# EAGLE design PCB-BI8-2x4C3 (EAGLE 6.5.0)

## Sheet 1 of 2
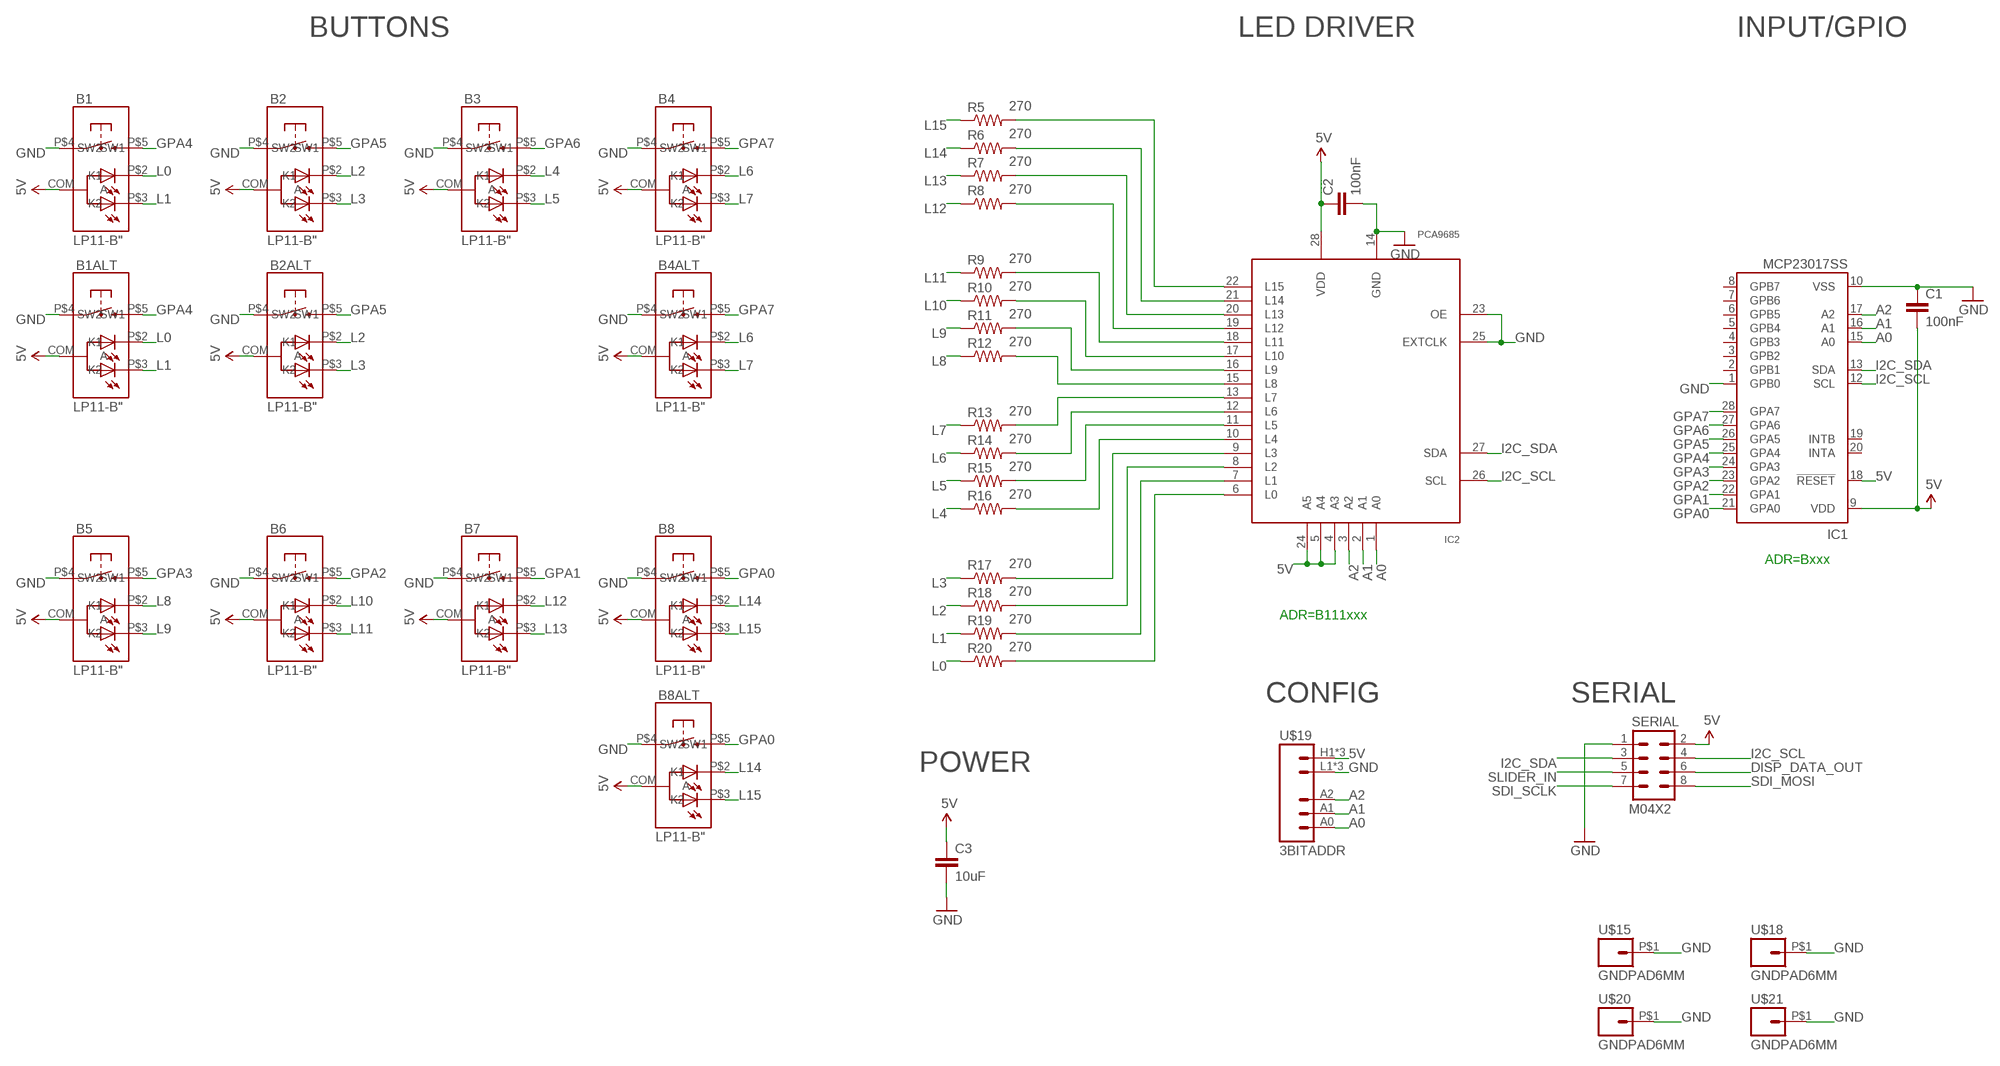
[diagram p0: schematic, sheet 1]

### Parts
B1  LP11-B"  [LP11]
B1ALT  LP11-B"  [LP11]
B2  LP11-B"  [LP11]
B2ALT  LP11-B"  [LP11]
B3  LP11-B"  [LP11]
B4  LP11-B"  [LP11]
B4ALT  LP11-B"  [LP11]
B5  LP11-B"  [LP11]
B6  LP11-B"  [LP11]
B7  LP11-B"  [LP11]
B8  LP11-B"  [LP11]
B8ALT  LP11-B"  [LP11]
C1  100nF  CAP0603-CAP  [0603-CAP]
C2  100nF  CAP0603-CAP  [0603-CAP]
C3  10uF  CAP0805  [0805]
IC1  MCP23017SS  [SSOP28]
IC2  PCA9685  [TSSOP28]
R5  270  RESISTOR0603-RES  [0603-RES]
R6  270  RESISTOR0603-RES  [0603-RES]
R7  270  RESISTOR0603-RES  [0603-RES]
R8  270  RESISTOR0603-RES  [0603-RES]
R9  270  RESISTOR0603-RES  [0603-RES]
R10  270  RESISTOR0603-RES  [0603-RES]
R11  270  RESISTOR0603-RES  [0603-RES]
R12  270  RESISTOR0603-RES  [0603-RES]
R13  270  RESISTOR0603-RES  [0603-RES]
R14  270  RESISTOR0603-RES  [0603-RES]
R15  270  RESISTOR0603-RES  [0603-RES]
R16  270  RESISTOR0603-RES  [0603-RES]
R17  270  RESISTOR0603-RES  [0603-RES]
R18  270  RESISTOR0603-RES  [0603-RES]
R19  270  RESISTOR0603-RES  [0603-RES]
R20  270  RESISTOR0603-RES  [0603-RES]
SERIAL  M04X2  [2X4]
U$15  GNDPAD6MM  [3.2MMPAD6MM]
U$18  GNDPAD6MM  [3.2MMPAD6MM]
U$19  3BITADDR  [3BITADDR]
U$20  GNDPAD6MM  [3.2MMPAD6MM]
U$21  GNDPAD6MM  [3.2MMPAD6MM]

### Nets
5V [Power]: B1.COM(A) B1ALT.COM(A) B2.COM(A) B2ALT.COM(A) B3.COM(A) B4.COM(A) B4ALT.COM(A) B5.COM(A) B6.COM(A) B7.COM(A) B8.COM(A) B8ALT.COM(A) C1.2 C2.1 C3.1 IC1.9(VDD) IC1.18(!RESET) IC2.4(A3) IC2.5(A4) IC2.24(A5) IC2.28(VDD) SERIAL.2 U$19.H1(VCC) U$19.H2(VCC) U$19.H3(VCC)
A0: IC1.15(A0) IC2.1(A0) U$19.A0
A1: IC1.16(A1) IC2.2(A1) U$19.A1
A2: IC1.17(A2) IC2.3(A2) U$19.A2
DISP_DATA_OUT: SERIAL.6
GND [Power]: B1.P$4(SW1) B1ALT.P$4(SW1) B2.P$4(SW1) B2ALT.P$4(SW1) B3.P$4(SW1) B4.P$4(SW1) B4ALT.P$4(SW1) B5.P$4(SW1) B6.P$4(SW1) B7.P$4(SW1) B8.P$4(SW1) B8ALT.P$4(SW1) C1.1 C2.2 C3.2 IC1.1(GPB0) IC1.10(VSS) IC2.14(GND) IC2.23(OE) IC2.25(EXTCLK) SERIAL.1 U$15.P$1 U$18.P$1 U$19.L1(GND) U$19.L2(GND) U$19.L3(GND) U$20.P$1 U$21.P$1
GPA0: B8.P$5(SW2) B8ALT.P$5(SW2) IC1.21(GPA0)
GPA1: B7.P$5(SW2) IC1.22(GPA1)
GPA2: B6.P$5(SW2) IC1.23(GPA2)
GPA3: B5.P$5(SW2) IC1.24(GPA3)
GPA4: B1.P$5(SW2) B1ALT.P$5(SW2) IC1.25(GPA4)
GPA5: B2.P$5(SW2) B2ALT.P$5(SW2) IC1.26(GPA5)
GPA6: B3.P$5(SW2) IC1.27(GPA6)
GPA7: B4.P$5(SW2) B4ALT.P$5(SW2) IC1.28(GPA7)
I2C_SCL: IC1.12(SCL) IC2.26(SCL) SERIAL.4
I2C_SDA: IC1.13(SDA) IC2.27(SDA) SERIAL.3
L0: B1.P$2(K1) B1ALT.P$2(K1) R20.1
L1: B1.P$3(K2) B1ALT.P$3(K2) R19.1
L2: B2.P$2(K1) B2ALT.P$2(K1) R18.1
L3: B2.P$3(K2) B2ALT.P$3(K2) R17.1
L4: B3.P$2(K1) R16.1
L5: B3.P$3(K2) R15.1
L6: B4.P$2(K1) B4ALT.P$2(K1) R14.1
L7: B4.P$3(K2) B4ALT.P$3(K2) R13.1
L8: B5.P$2(K1) R12.1
L9: B5.P$3(K2) R11.1
L10: B6.P$2(K1) R10.1
L11: B6.P$3(K2) R9.1
L12: B7.P$2(K1) R8.1
L13: B7.P$3(K2) R7.1
L14: B8.P$2(K1) B8ALT.P$2(K1) R6.1
L15: B8.P$3(K2) B8ALT.P$3(K2) R5.1
N$4: IC2.13(L7) R13.2
N$5: IC2.12(L6) R14.2
N$7: IC2.11(L5) R15.2
N$9: IC2.10(L4) R16.2
N$10: IC2.9(L3) R17.2
N$11: IC2.8(L2) R18.2
N$12: IC2.7(L1) R19.2
N$19: IC2.6(L0) R20.2
N$20: IC2.15(L8) R12.2
N$21: IC2.16(L9) R11.2
N$22: IC2.17(L10) R10.2
N$23: IC2.18(L11) R9.2
N$24: IC2.19(L12) R8.2
N$25: IC2.20(L13) R7.2
N$26: IC2.21(L14) R6.2
N$27: IC2.22(L15) R5.2
SDI_MOSI: SERIAL.8
SDI_SCLK: SERIAL.7
SLIDER_IN: SERIAL.5
Unconnected: IC1.2(GPB1) IC1.3(GPB2) IC1.4(GPB3) IC1.5(GPB4) IC1.6(GPB5) IC1.7(GPB6) IC1.8(GPB7) IC1.19(INTB) IC1.20(INTA)

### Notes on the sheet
- BUTTONS | LED DRIVER | INPUT/GPIO
- ADR=Bxxx
- ADR=B111xxx
- CONFIG | SERIAL
- POWER

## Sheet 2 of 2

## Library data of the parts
B1 B1ALT B2 B2ALT B3 B4 B4ALT B5-B8 B8ALT = SKAARHOJ:LP11-B
C1-C3 = SparkFun:CAP: Capacitor
IC1 = microchip:MCP23017: http://ww1.microchip.com/downloads/en/DeviceDoc/21952a.pdf Source: http://ww1.microchip.com/downloads/en/DeviceDoc/21952a.pdf; MF: MICROCHIP; MPN: MCP23017-E/SS; OC_FARNELL: 1467674; OC_NEWARK: 31K2960
IC2 = wsmith:PCA9685
R5-R20 = SparkFun:RESISTOR: Resistor
SERIAL = SparkFun:M04X2
U$15 U$18 U$20 U$21 = SKAARHOJ:GNDPAD
U$19 = SKAARHOJ:3BITADDR

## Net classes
0 default: width 0.203 mm, drill 0.406 mm, clearance 0.203 mm
1 Power: width 0.406 mm, drill 0.61 mm, clearance 0.203 mm

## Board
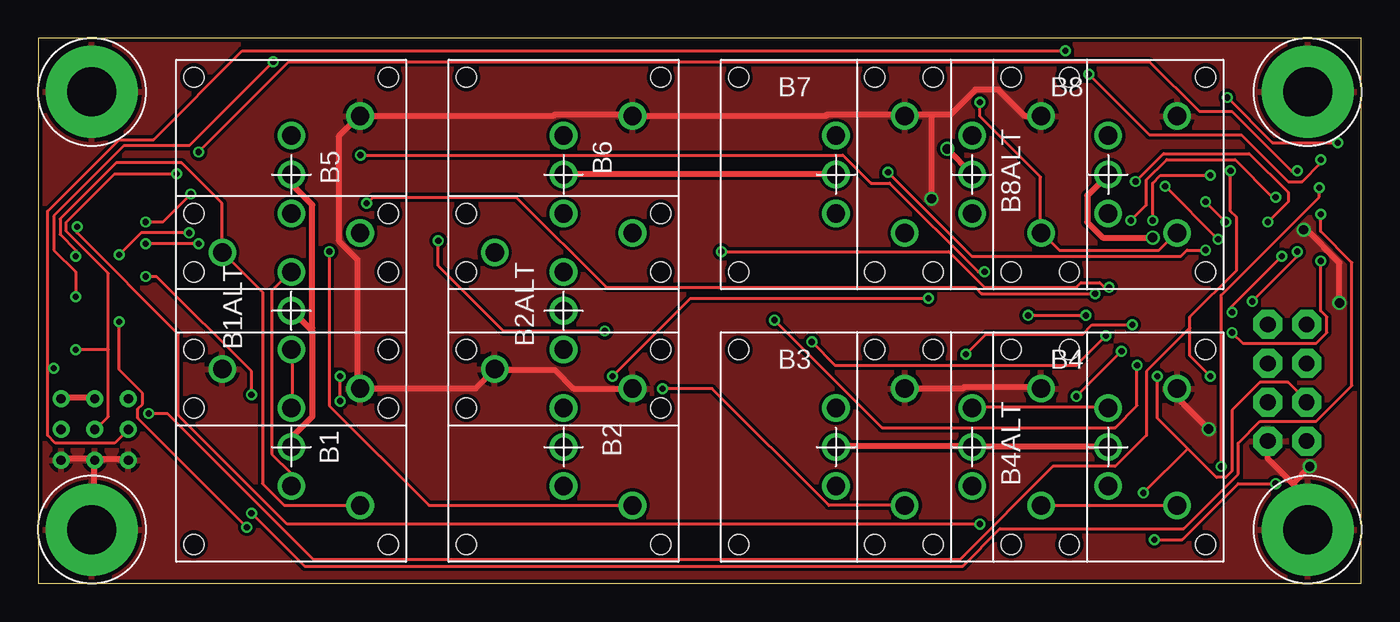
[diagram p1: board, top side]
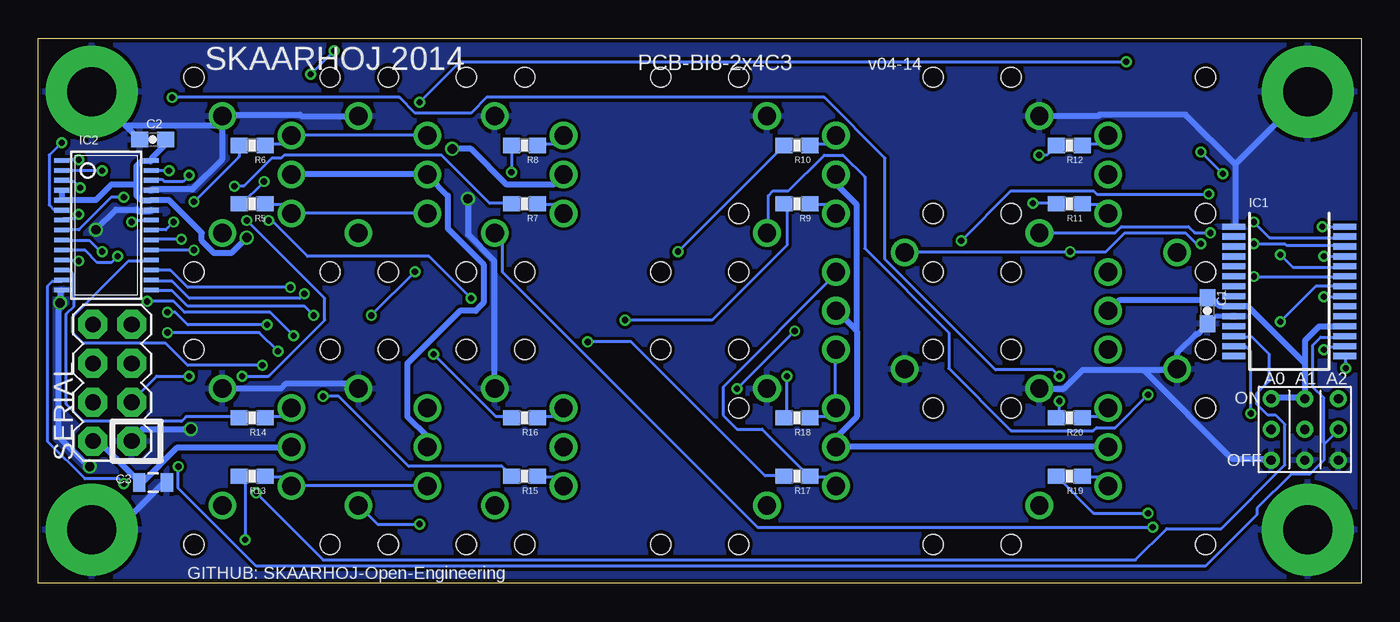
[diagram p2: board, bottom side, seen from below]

Size 86.36 x 35.56 mm. Coordinates in mm from the lower left corner, seen from the top.
Outline: 0,0 86.36,0 86.36,35.56 0,35.56 0,0
Copper layers (1*16): Top 0.035mm / dielectric 1.5mm / Bottom 0.035mm
Design rules "Fusion_eagle_rule_v1.1": minimum track width 6mil, minimum drill 12mil, track to track 6mil, track to pad 6mil, pad to pad 6mil, via to via 6mil, smd to smd 0mil, copper to edge 10mil, drill to drill 10mil, minimum pad ring 10mil, minimum via ring 6mil, stop-mask expansion 2mil, vias tented up to drill 100mil, thermal gap 10mil

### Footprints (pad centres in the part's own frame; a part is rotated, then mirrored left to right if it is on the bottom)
LP11 = drill 1.2: COM 0,0; P$2 0,2.54; P$3 0,-2.54; P$4 4.5,3.81; P$5 4.5,-3.81 | hole 1.3: -6.35,6.35; 6.35,6.35; 6.35,-6.35; -6.35,-6.35
0603-CAP = smd 1.1 x 1: 1 -0.85,0; 2 0.85,0
0805 = smd 0.8 x 1.2: 1 -0.9,0; 2 0.9,0
SSOP28 = smd 0.4 x 1.5: 1 -4.225,-3.625; 2 -3.575,-3.625; 3 -2.925,-3.625; 4 -2.275,-3.625; 5 -1.625,-3.625; 6 -0.975,-3.625; 7 -0.325,-3.625; 8 0.325,-3.625; 9 0.975,-3.625; 10 1.625,-3.625; 11 2.275,-3.625; 12 2.925,-3.625; 13 3.575,-3.625; 14 4.225,-3.625; 15 4.225,3.625; 16 3.575,3.625; 17 2.925,3.625; 18 2.275,3.625; 19 1.625,3.625; 20 0.975,3.625; 21 0.325,3.625; 22 -0.325,3.625; 23 -0.975,3.625; 24 -1.625,3.625; 25 -2.275,3.625; 26 -2.925,3.625; 27 -3.575,3.625; 28 -4.225,3.625
TSSOP28 = smd 0.305 x 0.991: 1 -4.225,-2.918; 2 -3.575,-2.918; 3 -2.925,-2.918; 4 -2.275,-2.918; 5 -1.625,-2.918; 6 -0.975,-2.918; 7 -0.325,-2.918; 8 0.325,-2.918; 9 0.975,-2.918; 10 1.625,-2.918; 11 2.275,-2.918; 12 2.925,-2.918; 13 3.575,-2.918; 14 4.225,-2.918; 15 4.225,2.918; 16 3.575,2.918; 17 2.925,2.918; 18 2.275,2.918; 19 1.625,2.918; 20 0.975,2.918; 21 0.325,2.918; 22 -0.325,2.918; 23 -0.975,2.918; 24 -1.625,2.918; 25 -2.275,2.918; 26 -2.925,2.918; 27 -3.575,2.918; 28 -4.225,2.918
0603-RES = smd 1.1 x 1: 1 -0.85,0; 2 0.85,0
2X4 = drill 1.016 pad 1.88 octagon: 1 -3.81,-1.27; 2 -3.81,1.27; 3 -1.27,-1.27; 4 -1.27,1.27; 5 1.27,-1.27; 6 1.27,1.27; 7 3.81,-1.27; 8 3.81,1.27
3.2MMPAD6MM = drill 3.2 pad 6: P$1 0,0
3BITADDR = drill 0.6: A0 -2.2,0; A1 0,0; A2 2.2,0; H1 -2.2,2; H2 0,2; H3 2.2,2; L1 -2.2,-2; L2 0,-2; L3 2.2,-2

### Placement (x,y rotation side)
B1  16.51,8.89 0 top
B1ALT  16.51,17.78 180 top
B2  34.29,8.89 0 top
B2ALT  34.29,17.78 180 top
B3  52.07,8.89 0 top
B4  69.85,8.89 0 top
B4ALT  60.96,8.89 0 top
B5  16.51,26.67 0 top
B6  34.29,26.67 0 top
B7  52.07,26.67 0 top
B8  69.85,26.67 0 top
B8ALT  60.96,26.67 0 top
C1  10.03,17.78 90 bottom
C2  78.89,28.96 180 bottom
C3  78.87,6.58 0 bottom
IC1  4.7,19.05 270 bottom
IC2  81.92,23.37 270 bottom
R5  72.39,24.77 180 bottom
R6  72.39,28.57 180 bottom
R7  54.61,24.77 180 bottom
R8  54.61,28.57 180 bottom
R9  36.83,24.77 180 bottom
R10  36.83,28.57 180 bottom
R11  19.05,24.77 180 bottom
R12  19.05,28.57 180 bottom
R13  72.39,6.99 180 bottom
R14  72.39,10.79 180 bottom
R15  54.61,6.99 180 bottom
R16  54.61,10.79 180 bottom
R17  36.83,6.99 180 bottom
R18  36.83,10.79 180 bottom
R19  19.05,6.99 180 bottom
R20  19.05,10.79 180 bottom
SERIAL  81.53,13.08 90 bottom
U$15  3.5,3.5 0 top
U$18  82.86,3.5 0 top
U$19  3.68,10.03 0 bottom
U$20  3.5,32.06 0 top
U$21  82.86,32.06 0 top

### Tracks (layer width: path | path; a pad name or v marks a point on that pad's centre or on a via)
5V  (via drill 0.61)
  Top 0.406: B3.COM 52.12,8.94 60.96,8.94 B4ALT.COM 61.06,8.94 69.8,8.94 B4.COM | U$19.H3 1.52,12.09 3.66,12.09 U$19.H2 | 17.78,16.56 16.56,17.78 B1ALT.COM | 17.78,16.56 17.88,16.46 17.88,10.87 16.56,9.55 16.56,8.94 B1.COM | B5.COM 16.56,26.62 16.56,26.01 17.88,24.69 17.88,16.66 17.78,16.56 | v72.75,22.55 69.49,22.55 68.48,23.57 68.48,25.3 B8.COM | B7.COM 52.02,26.72 34.34,26.72 B6.COM | v59.33,28.35 60.96,26.72 B8ALT.COM
  Bottom 0.406: SERIAL.2 82.8,9.25 82.4,9.25 79.86,6.71 79.86,6.6 C3.1 79.55,6.6 77.32,8.84 69.9,8.84 B4.COM | 3.66,14.43 3.66,12.09 U$19.H2 3.86,12.09 5.79,12.09 U$19.H1 | 3.66,14.43 3.66,15.85 2.74,16.76 1.12,16.76 IC1.18 | 3.66,14.43 3.76,14.43 7.42,18.09 8.13,18.09 IC1.9 8.33,18.09 9.25,18.09 9.75,18.59 9.96,18.59 C1.2 10.16,18.49 15.75,18.49 16.46,17.78 B1ALT.COM | IC2.4 84.84,25.6 IC2.5 84.63,24.99 82.6,24.99 81.58,26.01 79.96,26.01 | 79.96,26.01 79.96,27.23 79.65,27.53 79.05,27.53 IC2.28 78.94,27.74 78.13,28.55 78.13,28.96 C2.1 | 79.96,26.01 79.96,25.3 79.65,24.99 79.05,24.99 IC2.24 78.84,24.99 77.83,24.99 75.69,22.86 75.69,22.35 74.88,21.54 73.76,21.54 v72.75,22.55 | B8.COM 69.8,26.72 60.96,26.72 B8ALT.COM 60.86,26.52 59.64,25.3 59.64,23.16 57.3,20.83 57.3,18.29 57.81,17.78 58.83,17.78 62.28,14.33 62.28,10.87 60.96,9.55 B4ALT.COM | 33.02,16.56 34.24,17.78 B2ALT.COM | 33.02,16.56 32.92,16.46 32.92,10.87 34.24,9.55 34.24,8.94 B2.COM 34.14,8.94 16.56,8.94 B1.COM | B6.COM 34.24,26.62 34.24,26.01 32.92,24.69 32.92,16.66 33.02,16.56 | v59.33,28.35 58.12,28.35 55.78,26.01 52.73,26.01 B7.COM
A0  (via drill 0.41)
  Top 0.203: v83.72,27.64 83.72,27.43 82.5,26.21 81.58,26.21 78.54,29.26 72.54,29.26 v68.58,33.22 | v67.06,34.75 13.31,34.75 7.52,28.96 5.28,28.96 0.61,24.28 0.61,14.02 | 0.61,14.02 0.61,9.65 1.12,9.14 4.98,9.14 5.79,9.96 U$19.A0 | 0.61,14.02 v1.02,14.02
  Bottom 0.203: v83.72,27.64 84.73,27.64 IC2.1 | v67.06,34.75 v68.58,33.22 | v1.02,14.02 1.02,14.73 IC1.15
A1  (via drill 0.41)
  Top 0.203: v82.19,26.92 81.79,26.92 77.93,30.79 75.79,30.79 72.54,34.04 16.36,34.04 v10.46,28.14 | v9.04,26.72 4.98,26.72 1.83,23.57 1.83,22.96 4.57,20.22 4.57,15.24 | 4.57,15.24 4.57,10.87 3.76,10.06 U$19.A1 | 4.57,15.24 v2.44,15.24
  Bottom 0.203: v82.19,26.92 84.73,26.92 IC2.2 | v9.04,26.72 v10.46,28.14 | v2.44,15.24 2.23,15.44 1.12,15.44 IC1.16
A2  (via drill 0.41)
  Top 0.203: v83.62,25.81 83.62,25.2 77.22,18.8 v77.22,7.62
  Bottom 0.203: v83.62,25.81 84.02,26.21 84.73,26.21 IC2.3 | v77.22,7.62 77.22,6.2 72.14,1.12 10.16,1.12 6.81,4.47 6.81,4.88 4.57,7.11 3.35,7.11 2.44,8.03 2.44,9.04 2.39,9.09 | 2.39,9.09 1.52,9.96 U$19.A2 | IC1.17 1.12,16.05 2.64,16.05 3.15,15.54 3.15,12.8 2.44,12.09 2.44,9.14 2.39,9.09
GND  (via drill 0.61)
  Top 0.406: U$19.L3 1.52,8.13 3.66,8.13 U$19.L2 | U$19.L1 5.79,8.13 3.86,8.13 U$19.L2 | U$15.P$1 3.66,3.66 3.66,7.82 U$19.L2 | B2.P$4 34.95,12.7 33.73,13.92 29.97,13.92 B2ALT.P$4 29.77,13.92 28.55,12.7 B1.P$4 20.83,12.8 20.83,21.13 19.61,22.35 19.61,29.16 20.83,30.38 B5.P$4 33.63,30.48 33.73,30.58 38.61,30.58 B6.P$4 51.41,30.48 51.51,30.58 56.39,30.58 56.49,30.48 B7.P$4 56.69,30.58 58.32,30.58 | B3.P$4 60.35,12.7 60.45,12.8 65.33,12.8 65.43,12.7 B4ALT.P$4 | v82.6,23.06 82.8,23.06 84.94,20.93 v84.94,18.29 | SERIAL.1 80.26,8.13 81.89,6.5 | 81.89,6.5 82.8,5.59 82.8,3.56 U$18.P$1 | 81.89,6.5 v83.01,7.62 | v76.4,10.06 74.37,12.09 74.37,12.7 B4.P$4 | 58.32,30.58 59.54,30.58 61.16,32.21 62.69,32.21 64.41,30.48 B8ALT.P$4 | 58.32,30.58 v58.32,25.09
  Bottom 0.305: IC1.10 9.54,17.43 C1.1
  Bottom 0.406: C1.1 10.06,16.87 10.67,16.26 10.77,16.26 11.99,15.04 11.99,14.02 B1ALT.P$4 12.19,13.92 14.12,13.92 | 14.12,13.92 18.19,13.92 19.41,12.7 B1.P$4 | U$19.L1 5.89,8.13 8.43,8.13 14.12,13.82 14.12,13.92 | B4.P$4 70.51,12.7 70.21,13.01 65.84,13.01 65.53,12.7 B4ALT.P$4 | v82.6,23.06 81.28,24.38 79.96,24.38 79.86,24.28 79.05,24.28 IC2.23 | IC2.14 84.84,19.1 84.94,19 v84.94,18.29 85.04,18.19 85.04,9.55 83.11,7.62 v83.01,7.62 | C3.2 78.03,6.5 78.23,6.5 81.18,3.56 82.8,3.56 U$18.P$1 | v76.4,10.06 79.55,10.06 80.26,9.35 SERIAL.1 | 8.23,27.33 8.23,23.37 IC1.1 | U$20.P$1 8.23,27.33 | B5.P$4 17.17,30.48 17.07,30.58 11.48,30.58 8.23,27.33 | IC2.25 78.94,25.7 76.3,25.7 74.37,27.64 74.37,30.48 B8.P$4 | B8ALT.P$4 69.19,30.48 69.29,30.58 74.17,30.58 B8.P$4 | U$21.P$1 80.57,29.77 | 80.57,29.77 79.76,28.96 C2.2 | B8.P$4 74.47,29.87 80.47,29.87 80.57,29.77 | v58.32,25.09 58.32,22.76 56.59,21.03 56.59,12.7 B3.P$4
  pour Top: 0,0 86.36,0 86.36,35.56 0,35.56
  pour Bottom: 0,0 86.36,0 86.36,35.56 0,35.56
GPA0  (via drill 0.41)
  Top 0.203: v2.44,18.69 2.44,20.32 1.02,21.74 1.02,23.98 5.59,28.55 9.86,28.55 v15.34,34.04 | v61.47,31.39 61.47,30.48 65.43,26.52 65.43,22.86 B8ALT.P$5 65.53,22.86 66.65,21.74 73.15,21.74 74.27,22.86 B8.P$5
  Bottom 0.203: v2.44,18.69 1.12,18.69 IC1.21 | v15.34,34.04 58.83,34.04 v61.47,31.39
GPA1  (via drill 0.41)
  Top 0.203: v5.28,17.07 5.28,13.92 6.81,12.39 6.81,11.68 6.5,11.38 6.5,10.77 v13.61,3.66
  Bottom 0.203: v5.28,17.07 2.95,19.41 1.12,19.41 IC1.22 | v13.61,3.66 39.42,3.66 56.08,20.32 56.08,22.45 56.49,22.86 B7.P$5
GPA2  (via drill 0.41)
  Top 0.203: v7.01,20.02 7.72,20.02 13.92,13.82 v13.92,12.29
  Bottom 0.203: v7.01,20.02 1.12,20.02 IC1.23 | v13.92,12.29 16.05,10.16 17.27,10.16 17.48,9.96 22.86,9.96 26.92,14.02 26.92,16.36 32.41,21.84 32.41,26.52 33.83,27.94 35.05,27.94 37.39,25.6 38.41,25.6 38.71,25.3 38.71,22.86 B6.P$5
GPA3  (via drill 0.41)
  Top 0.203: v5.28,21.44 6.71,22.86 v9.86,22.86
  Bottom 0.203: v5.28,21.44 4.47,20.62 1.12,20.62 IC1.24 | v9.86,22.86 10.87,22.86 11.28,23.27 15.65,23.27 16.05,22.86 B5.P$5
GPA4  (via drill 0.41)
  Top 0.203: v2.44,21.34 2.44,21.74 1.42,22.76 1.42,23.77 5.08,27.43 9.35,27.43 11.99,24.79 11.99,21.64 B1ALT.P$5 12.09,21.54 14.63,19 14.63,6.5 16.05,5.08 B1.P$5
  Bottom 0.203: v2.44,21.34 1.12,21.34 IC1.25
GPA5  (via drill 0.41)
  Top 0.203: v10.46,22.15 v7.01,22.15 | B2.P$5 25.5,5.08 19,11.58 v19,21.64
  Bottom 0.203: v7.01,22.15 4.98,22.15 4.88,22.05 1.12,22.05 IC1.26 | v10.46,22.15 10.77,22.15 11.48,22.86 15.44,22.86 16.66,21.64 v19,21.64 29.77,21.64 B2ALT.P$5
GPA6  (via drill 0.41)
  Top 0.203: v7.01,23.57 8.13,23.57 v9.96,25.4 | v26.11,22.35 26.11,20.73 30.38,16.46 v36.98,16.46 | v40.74,12.7 43.99,12.7 51.61,5.08 B3.P$5
  Bottom 0.203: v7.01,23.57 5.99,22.55 1.12,22.55 IC1.27 | v9.96,25.4 17.27,25.4 17.48,25.6 22.86,25.6 v26.11,22.35 | v40.74,12.7 v36.98,16.46
GPA7  (via drill 0.41)
  Top 0.203: v2.54,23.27 2.54,22.86 9.14,16.26 9.14,10.97 16.26,3.86 v61.47,3.86 | B4ALT.P$5 B4.P$5
  Bottom 0.203: v2.54,23.27 1.12,23.27 IC1.28 | v61.47,3.86 64.21,3.86 65.43,5.08 B4ALT.P$5
I2C_SCL  (via drill 0.41)
  Top 0.203: v76.5,26.62 73.25,26.62 72.75,26.11 v72.75,23.67 | v73.05,13.51 73.05,10.77 75.03,8.79 | 75.03,8.79 76.91,6.91 77.52,6.91 77.93,7.32 77.93,11.28 79.76,13.11 81.58,13.11 82.8,11.89 SERIAL.4 | 75.03,8.79 v72.14,5.89
  Bottom 0.203: v76.5,26.62 76.91,26.21 78.13,26.21 78.23,26.31 78.94,26.31 IC2.26 | v72.75,23.67 67.67,18.59 67.67,17.17 71.32,13.51 v73.05,13.51 | v72.14,5.89 67.77,1.52 14.73,1.52 12.7,3.56 9.14,3.56 4.98,7.72 4.98,10.36 5.59,10.97 6.1,10.97 6.81,11.68 6.81,12.39 5.99,13.21 5.99,14.94 7.11,16.05 8.23,16.05 IC1.12
I2C_SDA  (via drill 0.41)
  Top 0.203: v77.83,26.92 77.83,24.28 78.23,23.88 78.23,20.42 75.18,17.37 75.18,16.66 | 75.18,16.66 75.18,14.83 v76.5,13.51 | v7.21,11.07 8.43,11.07 17.98,1.52 60.15,1.52 66.24,7.62 70.31,7.62 72.34,9.65 72.34,13.82 75.18,16.66
  Bottom 0.203: v77.83,26.92 78.94,26.92 IC2.27 | v76.5,13.51 78.64,13.51 80.26,11.89 SERIAL.3 | v7.21,11.07 7.21,15.14 7.52,15.44 8.23,15.44 IC1.13
L0
  Top 0.203: B1.P$2 16.56,11.48 16.56,15.24 B1ALT.P$2
  Bottom 0.203: B1.P$2 17.07,10.87 18.19,10.87 R20.1
L1
  Top 0.203: B1.P$3 16.46,6.4 16.46,7.21 15.24,8.43 15.24,19.1 16.46,20.32 B1ALT.P$3
  Bottom 0.203: B1.P$3 17.07,6.91 18.19,6.91 R19.1
L2
  Bottom 0.203: R18.1 35.97,10.87 34.85,10.87 B2.P$2 34.34,11.48 34.34,15.24 B2ALT.P$2
L3
  Bottom 0.203: B2.P$3 34.85,6.91 35.97,6.91 R17.1 36.07,7.01 39.12,10.06 40.74,10.06 41.66,10.97 41.66,12.8 34.34,20.12 34.34,20.32 B2ALT.P$3
L4
  Bottom 0.203: B3.P$2 52.63,10.87 53.75,10.87 R16.1
L5
  Bottom 0.203: B3.P$3 52.63,6.91 53.75,6.91 R15.1
L6
  Top 0.203: B4ALT.P$2 60.96,11.48 69.8,11.48 B4.P$2
  Bottom 0.203: B4.P$2 70.41,10.87 71.53,10.87 R14.1
L7
  Bottom 0.203: R13.1 71.53,6.91 70.41,6.91 B4.P$3 69.8,6.4 60.96,6.4 B4ALT.P$3
L8
  Bottom 0.203: B5.P$2 17.07,28.65 18.19,28.65 R12.1
L9
  Bottom 0.203: B5.P$3 17.07,24.69 18.19,24.69 R11.1
L10
  Bottom 0.203: B6.P$2 34.85,28.65 35.97,28.65 R10.1
L11
  Bottom 0.203: B6.P$3 34.85,24.69 35.97,24.69 R9.1
L12
  Bottom 0.203: B7.P$2 52.63,28.65 53.75,28.65 R8.1
L13
  Bottom 0.203: B7.P$3 52.63,24.69 53.75,24.69 R7.1
L14
  Bottom 0.203: R6.1 71.53,28.65 70.41,28.65 B8.P$2 69.8,29.26 60.96,29.26 B8ALT.P$2
L15
  Bottom 0.203: R5.1 71.53,24.69 70.41,24.69 B8.P$3 69.8,24.18 60.96,24.18 B8ALT.P$3
N$4  (via drill 0.41)
  Top 0.203: v80.77,6.5 78.33,6.5 74.68,2.85 v72.85,2.85
  Bottom 0.203: v80.77,6.5 81.08,6.81 83.31,6.81 85.75,9.25 85.75,19.41 85.45,19.71 84.84,19.71 IC2.13 | v72.85,2.85 72.85,6.6 73.15,6.91 R13.2
N$5
  Bottom 0.203: IC2.12 84.73,20.42 84.33,20.42 84.02,20.12 84.02,18.09 84.53,17.58 84.53,11.68 83.41,10.57 77.01,10.57 76.71,10.87 73.25,10.87 R14.2
N$7  (via drill 0.41)
  Top 0.203: v83.72,21.03 83.72,17.78 84.12,17.37 84.12,16.36 83.41,15.65 78.64,15.65 v77.93,16.36 | v67.77,12.19 v70.71,15.14
  Bottom 0.203: v83.72,21.03 84.73,21.03 IC2.11 | v77.93,16.36 71.93,16.36 v70.71,15.14 | v67.77,12.19 66.75,12.19 62.18,7.62 56.08,7.62 55.47,7.01 R15.2
N$9  (via drill 0.41)
  Top 0.203: v81.18,21.34 77.93,18.09 v77.93,17.68 | v71.42,16.87 68.78,16.87 68.17,16.26 61.87,16.26 v60.55,14.94
  Bottom 0.203: v81.18,21.34 81.58,20.93 82.5,20.93 83.31,21.74 84.73,21.74 IC2.10 | v77.93,17.68 77.42,17.68 76.61,16.87 v71.42,16.87 | v60.55,14.94 56.49,10.87 55.47,10.87 R16.2
N$10  (via drill 0.41)
  Top 0.203: v82.19,21.64 82.19,21.34 v79.25,18.39 | v69.7,16.15 67.77,14.22 52.02,14.22 v50.49,15.75
  Bottom 0.203: v82.19,21.64 82.3,21.64 83.01,22.35 84.73,22.35 IC2.9 | v79.25,18.39 77.52,18.39 76.81,17.68 71.22,17.68 v69.7,16.15 | v50.49,15.75 47.65,15.75 38.91,7.01 37.69,7.01 R17.2
N$11  (via drill 0.41)
  Top 0.203: v80.77,25.2 80.57,25.2 78.13,27.64 73.66,27.64 72.34,26.31 72.34,24.69 v71.32,23.67 | v58.12,18.59 42.57,18.59 v37.49,13.51
  Bottom 0.203: v80.77,25.2 81.58,25.2 83.72,23.06 84.73,23.06 IC2.8 | v71.32,23.67 71.12,23.67 68.78,21.34 60.86,21.34 v58.12,18.59 | v37.49,13.51 37.49,10.97 37.59,10.87 R18.2
N$12  (via drill 0.41)
  Top 0.203: v83.72,24.08 83.72,22.96 85.75,20.93 85.75,12.9 83.41,10.57 79.76,10.57 78.33,9.14 78.33,7.11 74.78,3.56 62.79,3.56 60.35,1.12 17.37,1.12 v13.92,4.57
  Bottom 0.203: v83.72,24.08 84.02,23.77 84.73,23.77 IC2.7 | v13.92,4.57 17.48,4.57 19.81,6.91 R19.2
N$19  (via drill 0.41)
  Top 0.203: v84.84,28.75 80.57,28.75 v77.62,31.7 | v19.71,11.89 v19.71,13.51
  Bottom 0.203: v84.84,28.75 85.65,27.94 85.65,24.69 85.34,24.38 84.84,24.38 IC2.6 | v77.62,31.7 62.79,31.7 61.77,30.68 58.12,30.68 57.1,31.7 35.05,31.7 31.09,27.74 31.09,21.13 23.88,13.92 20.12,13.92 v19.71,13.51 | v19.71,11.89 19.71,10.97 19.81,10.87 R20.2
N$20  (via drill 0.41)
  Top 0.203: v64.62,17.48 v68.38,17.48 | v61.77,20.32 61.37,20.32 55.58,26.11 54.36,26.11 52.53,27.94 v21.03,27.94
  Bottom 0.203: v68.38,17.48 68.99,18.09 76.61,18.09 77.62,19.1 78.94,19.1 IC2.15 | v61.77,20.32 v64.62,17.48 | v21.03,27.94 20.52,27.94 19.91,28.55 R12.2
N$21  (via drill 0.41)
  Top 0.203: v68.99,18.9 61.57,18.9 61.16,19.3 37.08,19.3 31.19,25.2 21.84,25.2 v21.44,24.79
  Bottom 0.203: v68.99,18.9 69.29,18.59 76.5,18.59 77.62,19.71 78.94,19.71 IC2.16 | v21.44,24.79 19.91,24.79 R11.2
N$22  (via drill 0.41)
  Top 0.203: v69.9,19.3 69.6,19.3 69.29,19.61 68.07,19.61 67.77,19.3 61.77,19.3 59.44,21.64 v44.6,21.64
  Bottom 0.203: v69.9,19.3 76.61,19.3 77.72,20.42 78.94,20.42 IC2.17 | v44.6,21.64 37.69,28.55 R10.2
N$23  (via drill 0.41)
  Top 0.203: v71.73,14.22 71.73,11.58 70.31,10.16 55.07,10.16 v48.06,17.17
  Bottom 0.203: v71.73,14.22 76.61,14.22 78.03,15.65 83.41,15.65 84.12,16.36 84.12,17.37 80.47,21.03 79.05,21.03 IC2.18 | v48.06,17.17 42.37,17.17 37.49,22.05 37.49,24.59 37.59,24.69 R9.2
N$24  (via drill 0.41)
  Top 0.203: v76.2,21.74 74.98,21.74 74.57,21.34 60.96,21.34 v55.47,26.82
  Bottom 0.203: v76.2,21.74 78.94,21.74 IC2.19 | v55.47,26.82 55.47,28.55 R8.2
N$25  (via drill 0.41)
  Top 0.203: v73.56,25.91 v77.01,22.45
  Bottom 0.203: v77.01,22.45 78.94,22.45 IC2.20 | v73.56,25.91 72.95,25.91 71.12,27.74 70.51,27.74 70.31,27.94 60.05,27.94 56.9,24.79 55.47,24.79 R7.2
N$26  (via drill 0.41)
  Top 0.203: v76.2,24.89 v77.52,23.57
  Bottom 0.203: v77.52,23.57 78.03,23.06 78.94,23.06 IC2.21 | v76.2,24.89 73.25,27.84 73.25,28.55 R6.2
N$27  (via drill 0.41)
  Top 0.203: v80.26,23.57 81.58,24.89 81.58,25.5 79.05,28.04 73.46,28.04 v71.63,26.21
  Bottom 0.203: v80.26,23.57 80.16,23.67 79.05,23.67 IC2.22 | v71.63,26.21 73.15,24.69 R5.2

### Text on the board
_bsilk: v04-14 | PCB-BI8-2x4C3 | SKAARHOJ 2014 | GITHUB: SKAARHOJ-Open-Engineering

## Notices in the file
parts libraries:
SparkFun: Licensing: CC v3.0 Share-Alike You are welcome to use this library for commercial purposes.
